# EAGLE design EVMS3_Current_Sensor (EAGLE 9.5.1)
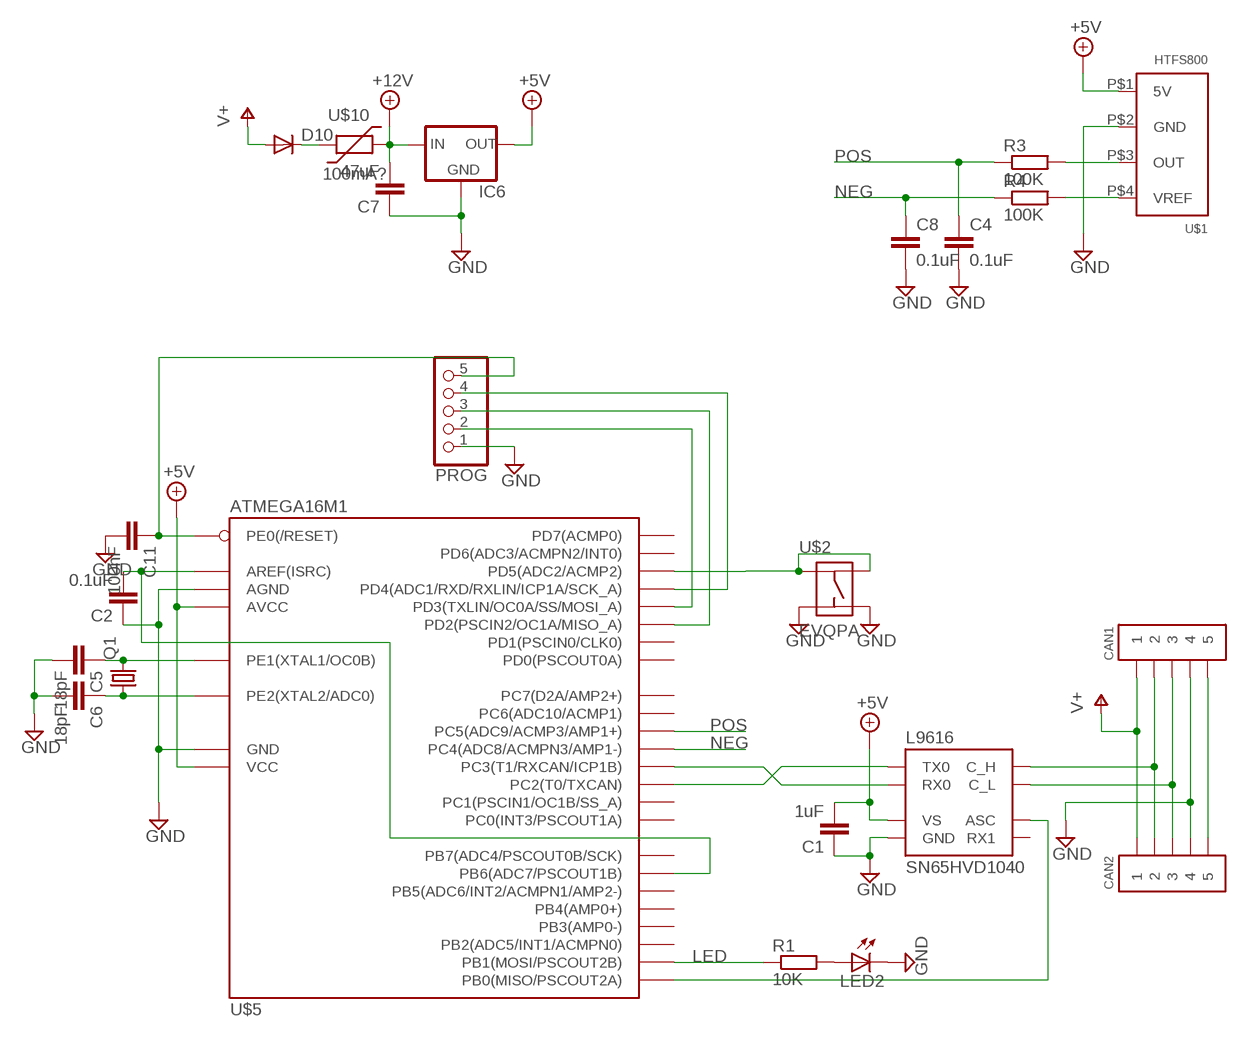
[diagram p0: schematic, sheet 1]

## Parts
C1  1uF  C-EUC1206  [C1206]
C2  0.1uF  C-EUC1206  [C1206]
C4  0.1uF  C-EUC1206  [C1206]
C5  18pF  C-EUC0805  [C0805]
C6  18pF  C-EUC0805  [C0805]
C7  47uF  C-EUC1206  [C1206]
C8  0.1uF  C-EUC1206  [C1206]
C11  100nF  C-EUC1206  [C1206]
CAN1  MOLEX-39502-1005  [MOLEX-39502-1005]
CAN2  MOLEX-39502-1005  [MOLEX-39502-1005]
D10  DIODE-SOD123  [SOD123]
IC6  78LXXSOT89  [SOT89R]
LED2  LED3MM  [LED3MM]
PROG  PINHD-1X5  [1X05]
Q1  CRYSTALCTS406  [CTS406]
R1  10K  R-EU_R1206  [R1206]
R3  100K  R-EU_R1206  [R1206]
R4  100K  R-EU_R1206  [R1206]
SN65HVD1040  L9616  [SOIC8]
U$1  HTFS800  [HTFS800]
U$2  EVQPA  [EVQPA]
U$5  ATMEGA16M1  [TQFP32]
U$10  100mA?  1206_POLYSWITCH  [1206]

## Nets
+5V: C1.2 IC6.2(OUT) SN65HVD1040.P$3(VS) U$1.P$1(5V) U$5.4(VCC) U$5.19(AVCC)
+12V: C7.2 IC6.1(IN) U$10.P$2
BUTTON: U$2.B U$2.B2 U$5.13(PD5(ADC2/ACMP2))
GND: C1.1 C2.1 C4.2 C5.2 C6.2 C7.1 C8.2 C11.2 CAN1.4 CAN2.4 IC6.4(GND) LED2.K(C) PROG.1 SN65HVD1040.P$2(GND) U$1.P$2(GND) U$2.A U$2.A2 U$5.5(GND) U$5.20(AGND)
LED: R1.1 U$5.9(PB1(MOSI/PSCOUT2B))
N$1: LED2.A R1.2
N$2: CAN1.5 CAN2.5
N$3: SN65HVD1040.P$8(ASC) U$5.8(PB0(MISO/PSCOUT2A))
N$4: R3.2 U$1.P$3(OUT)
N$5: R4.2 U$1.P$4(VREF)
N$7: CAN1.2 CAN2.2 SN65HVD1040.P$7(C_H)
N$10: CAN1.3 CAN2.3 SN65HVD1040.P$6(C_L)
N$12: SN65HVD1040.P$1(TX0) U$5.6(PC2(T0/TXCAN))
N$15: D10.C U$10.P$1
N$17: SN65HVD1040.P$4(RX0) U$5.7(PC3(T1/RXCAN/ICP1B))
N$21: C6.1 Q1.1 U$5.11(PE2(XTAL2/ADC0))
N$34: C5.1 Q1.3 U$5.10(PE1(XTAL1/OC0B))
N$42: C2.2 U$5.21(AREF(ISRC)) U$5.27(PB6(ADC7/PSCOUT1B))
N$44: C11.1 PROG.5 U$5.31(PE0(/RESET))
NEG: C8.1 R4.1 U$5.17(PC4(ADC8/ACMPN3/AMP1-))
OUT1: PROG.2 U$5.2(PD3(TXLIN/OC0A/SS/MOSI_A))
OUT2: PROG.3 U$5.1(PD2(PSCIN2/OC1A/MISO_A))
OUT3: PROG.4 U$5.12(PD4(ADC1/RXD/RXLIN/ICP1A/SCK_A))
POS: C4.1 R3.1 U$5.18(PC5(ADC9/ACMP3/AMP1+))
V+: CAN1.1 CAN2.1 D10.A
Unconnected: SN65HVD1040.P$5(RX1) U$5.3(PC1(PSCIN1/OC1B/SS_A)) U$5.14(PD6(ADC3/ACMPN2/INT0)) U$5.15(PD7(ACMP0)) U$5.16(PB2(ADC5/INT1/ACMPN0)) U$5.22(PC6(ADC10/ACMP1)) U$5.23(PB3(AMP0-)) U$5.24(PB4(AMP0+)) U$5.25(PC7(D2A/AMP2+)) U$5.26(PB5(ADC6/INT2/ACMPN1/AMP2-)) U$5.28(PB7(ADC4/PSCOUT0B/SCK)) U$5.29(PD0(PSCOUT0A)) U$5.30(PC0(INT3/PSCOUT1A)) U$5.32(PD1(PSCIN0/CLK0))

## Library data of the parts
C1 C2 C4-C8 C11 = resistor:C-EU: CAPACITOR, European symbol
CAN1 CAN2 = Ians parts:MOLEX-39502-1005
D10 = diode:DIODE-: DIODE
IC6 = v-reg:78LXX: VOLTAGE REGULATOR
LED2 = led:LED: LED
PROG = pinhead:PINHD-1X5: PIN HEADER
Q1 = crystal:CRYSTAL: CRYSTAL
R1 R3 R4 = resistor:R-EU_: RESISTOR, European symbol
SN65HVD1040 = Ians parts:L9616
U$1 = Ians parts:HTFS800
U$2 = Ians parts:EVQPA
U$5 = Ians parts:ATMEGA16M1
U$10 = Ians parts:1206_POLYSWITCH

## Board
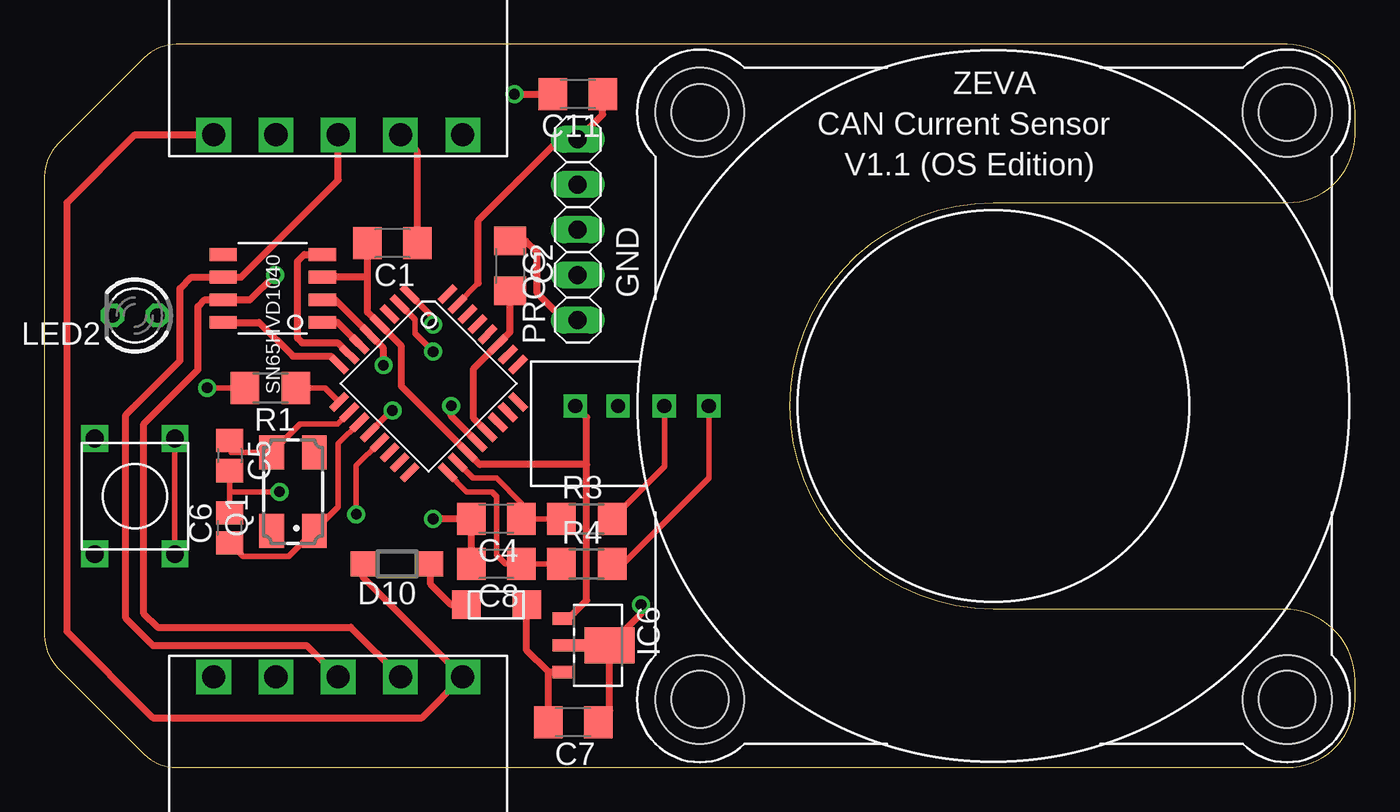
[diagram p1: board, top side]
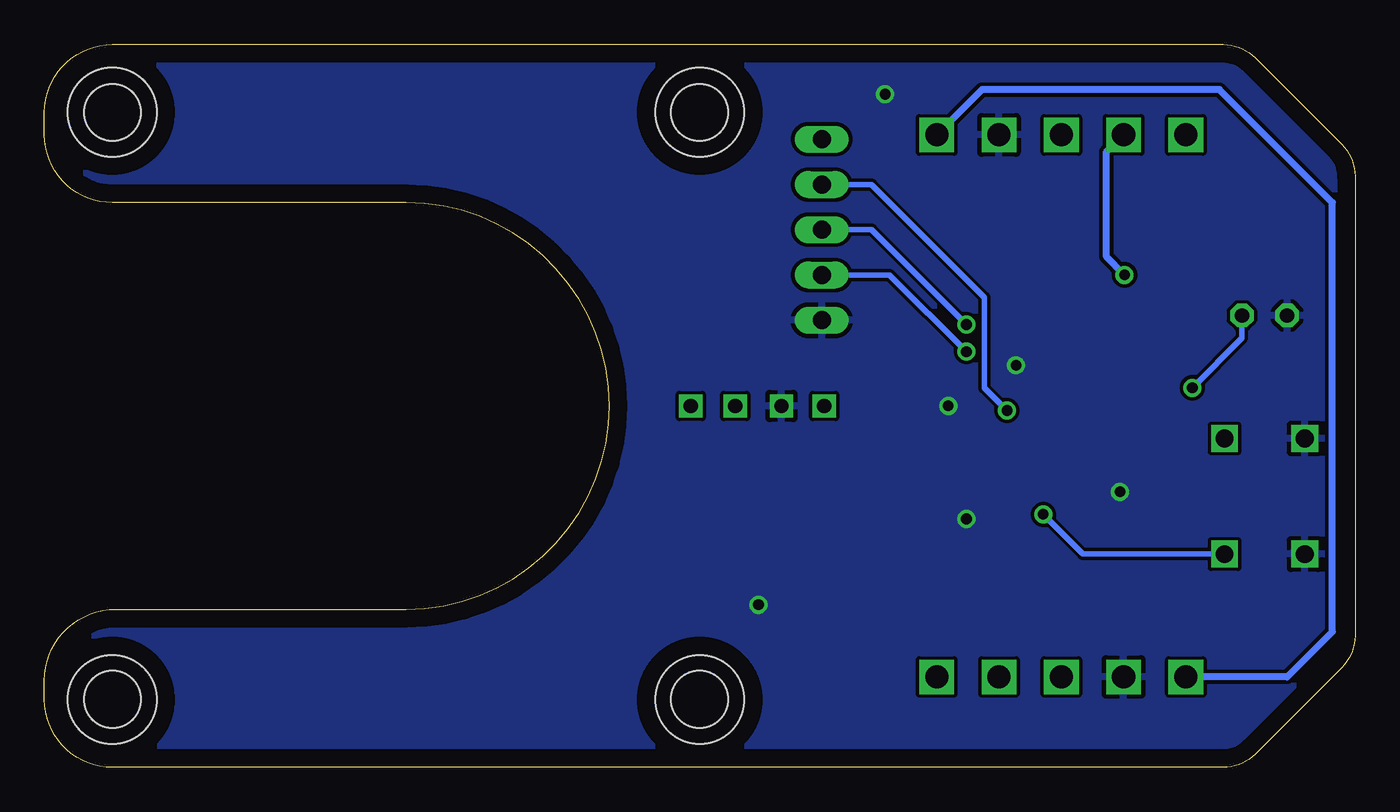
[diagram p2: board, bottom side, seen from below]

Size 73.66 x 40.64 mm. Coordinates in mm from the lower left corner, seen from the top.
Outline: 53.34,8.89 arc-90 41.91,20.32 arc-90 53.34,31.75 69.85,31.75 arc90 73.66,35.56 73.66,36.83 arc90 69.85,40.64 7.4,40.64 arc45 5.61,39.9 0.74,35.03 arc45 0,33.24 0,7.4 arc45 0.74,5.61 5.61,0.74 arc45 7.4,0 69.85,0 arc90 73.66,3.81 73.66,4.87 arc90 69.64,8.89 53.34,8.89
Copper layers (1*16): Top 0.035mm / dielectric 1.5mm / Bottom 0.035mm
Design rules "default *": minimum track width 10mil, minimum drill 20mil, track to track 8mil, track to pad 8mil, pad to pad 8mil, via to via 8mil, smd to smd 8mil, copper to edge 40mil, drill to drill 8mil, minimum pad ring 10mil, minimum via ring 8mil, stop-mask expansion 4mil, vias tented up to drill 0mil, thermal gap 10mil
Holes 5 mm at 36.83,36.83 69.85,36.83 36.83,3.81 69.85,3.81

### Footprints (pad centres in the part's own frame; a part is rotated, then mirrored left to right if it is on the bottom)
C1206 = smd 1.6 x 1.8: 1 -1.4,0; 2 1.4,0
C0805 = smd 1.3 x 1.5: 1 -0.85,0; 2 0.85,0
MOLEX-39502-1005 = drill 1.3 square: 1 -7,0; 2 -3.5,0; 3 0,0; 4 3.5,0; 5 7,0
SOD123 = smd 1.4 x 1.4: A 1.9,0; C -1.9,0
SOT89R = smd 0.7 x 1.1: 1 1.5,-1.75; 2 -1.5,-1.75 | smd 0.7 x 1.8: 3 0,-1.4 | smd 2 x 2.8: 4 0,0.9
LED3MM = drill 0.813 octagon: A -1.27,0; K 1.27,0
1X05 = drill 1.016 long: 1 -5.08,0; 2 -2.54,0; 3 0,0; 4 2.54,0; 5 5.08,0
CTS406 = smd 1.9 x 1.4: 1 -2.2,-1.2; 2 2.2,-1.2; 3 2.2,1.2; 4 -2.2,1.2
R1206 = smd 1.6 x 1.803: 1 -1.422,0; 2 1.422,0
SOIC8 = smd 1.524 x 0.711: P$1 -2.794,1.905; P$2 -2.794,0.635; P$3 -2.794,-0.635; P$4 -2.794,-1.905; P$5 2.794,-1.905; P$6 2.794,-0.635; P$7 2.794,0.635; P$8 2.794,1.905
HTFS800 = drill 0.8 square: P$1 0,-23.5; P$2 0,-21.1; P$3 0,-18.5; P$4 0,-16 | hole 3.2: -16.5,16.5; 16.5,16.5; 16.5,-16.5; -16.5,-16.5
EVQPA = drill 1 square: A -2.25,3.25; A2 -2.25,-3.25; B 2.25,3.25; B2 2.25,-3.25
TQFP32 = smd 1.2 x 0.4: 1 -4.3,2.8; 2 -4.3,2; 3 -4.3,1.2; 4 -4.3,0.4; 5 -4.3,-0.4; 6 -4.3,-1.2; 7 -4.3,-2; 8 -4.3,-2.8; 17 4.3,-2.8; 18 4.3,-2; 19 4.3,-1.2; 20 4.3,-0.4; 21 4.3,0.4; 22 4.3,1.2; 23 4.3,2; 24 4.3,2.8 | smd 0.4 x 1.2: 9 -2.8,-4.3; 10 -2,-4.3; 11 -1.2,-4.3; 12 -0.4,-4.3; 13 0.4,-4.3; 14 1.2,-4.3; 15 2,-4.3; 16 2.8,-4.3; 25 2.8,4.3; 26 2,4.3; 27 1.2,4.3; 28 0.4,4.3; 29 -0.4,4.3; 30 -1.2,4.3; 31 -2,4.3; 32 -2.8,4.3
1206 = smd 1.6 x 1.6: P$1 -1.7,0; P$2 1.7,0

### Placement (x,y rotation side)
C1  19.56,29.46 180 top
C2  26.16,28.19 270 top
C4  25.4,13.97 180 top
C5  10.41,17.53 270 top
C6  10.41,13.46 90 top
C7  29.72,2.54 180 top
C8  25.4,11.43 180 top
C11  29.97,37.85 180 top
CAN1  16.51,35.56 0 top
CAN2  16.51,5.08 180 top
D10  19.81,11.43 180 top
IC6  30.86,6.86 270 top
LED2  5.08,25.4 180 top
PROG  29.97,30.23 90 top
Q1  13.97,15.49 90 top
R1  12.7,21.34 180 top
R3  30.48,13.97 0 top
R4  30.48,11.43 0 top
SN65HVD1040  12.83,26.92 180 top
U$1  53.34,20.32 270 top
U$2  5.08,15.24 0 top
U$5  21.59,21.59 315 top
U$10  25.4,9.14 0 top

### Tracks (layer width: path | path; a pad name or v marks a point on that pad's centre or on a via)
+5V
  Top 0.406: IC6.2 29.44,8.36 30.48,9.4 30.48,17.02 | 30.48,17.02 30.48,19.68 U$1.P$1 | 30.48,17.02 24.46,17.02 U$5.19 20.07,21.42 20.07,23.68 U$5.4 18.16,25.59 18.16,27.56 | 18.16,27.56 C1.2 | 18.16,27.56 SN65HVD1040.P$3
+12V
  Top 0.406: 28.76,5.46 IC6.1 28.32,5.36 | C7.2 28.32,5.36 | U$10.P$2 27.1,6.58 28.32,5.36
BUTTON  (via drill 0.6)
  Top 0.305: U$2.B2 U$2.B | U$5.13 17.53,16.96 v17.53,14.22
  Bottom 0.305: U$2.B2 15.29,11.99 v17.53,14.22
GND  (via drill 0.6)
  Top 0.305: C6.2 10.41,15.49 | 10.41,15.49 C5.2 | 10.41,15.49 v13.21,15.49
  Top 0.406: v21.84,13.97 C4.2 C8.2 | U$5.20 22.86,19.75 v22.86,20.32 | v19.05,22.61 19.05,23.56 U$5.5 16.32,26.29 SN65HVD1040.P$2 | C2.1 27.05,29.59 27.69,28.96 27.69,26.67 29.21,25.15 PROG.1 | v26.42,37.85 C11.2 | C1.1 20.96,34.61 CAN1.4 | C7.1 31.76,3.18 IC6.4 33.53,8.62 v33.53,9.14
  pour Bottom: -1.27,-0.64 74.93,-0.64 74.93,41.27 -1.27,41.27
LED
  Top 0.305: R1.1 15.76,21.34 U$5.9
N$1  (via drill 0.6)
  Top 0.305: v9.14,21.34 R1.2
  Bottom 0.305: LED2.A 6.35,24.13 v9.14,21.34
N$2
  Bottom 0.406: CAN2.5 3.81,5.08 1.27,7.62 1.27,31.75 7.62,38.1 20.97,38.1 CAN1.5
N$3
  Top 0.406: U$5.8 16.11,23.11 13.97,23.11 12.06,25.02 SN65HVD1040.P$8
N$4
  Top 0.305: U$1.P$3 34.84,16.91 R3.2
N$5
  Top 0.305: U$1.P$4 37.34,16.26 32.51,11.43 R4.2
N$7  (via drill 0.6)
  Top 0.406: v12.95,27.69 11.56,26.29 SN65HVD1040.P$7 9.02,26.29 8.64,25.91 8.64,22.35 5.59,19.3 5.59,8.64 6.35,7.87 17.22,7.87 CAN2.2
  Bottom 0.406: v12.95,27.69 13.97,28.7 13.97,34.6 CAN1.2
N$10
  Top 0.406: CAN1.3 16.51,33.02 11.05,27.56 SN65HVD1040.P$6 8.26,27.56 7.62,26.92 7.62,22.86 4.57,19.81 4.57,8.38 6.1,6.86 14.73,6.86 CAN2.3
N$12
  Top 0.406: SN65HVD1040.P$1 16.46,25.02 U$5.6
N$15
  Top 0.406: D10.C 21.71,10.29 22.86,9.14 U$10.P$1
N$17
  Top 0.406: U$5.7 16.48,23.88 14.48,23.88 14.22,24.13 14.22,28.45 14.61,28.83 SN65HVD1040.P$4
N$21
  Top 0.305: U$5.11 16.51,18.21 16.51,14.63 Q1.1 13.73,11.85 11.18,11.85 C6.1
N$34
  Top 0.305: U$5.10 16.48,19.3 14.38,19.3 Q1.3 10.49,17.69 C5.1
N$42
  Top 0.406: U$5.21 24.13,19.62 24.13,22.43 U$5.27 26.16,24.46 C2.2
N$44
  Top 0.305: U$5.31 24.38,27.21
  Top 0.406: 24.38,27.21 24.38,30.73 28.96,35.31 PROG.5 31.37,36.71 C11.1
NEG
  Top 0.305: R4.1 C8.1 25.91,11.43 25.4,11.94 25.4,15.24 25.15,15.49 23.73,15.49 U$5.17
OUT1  (via drill 0.6)
  Top 0.305: U$5.2 20.83,25.18 20.83,24.38 v21.84,23.37
  Bottom 0.305: PROG.2 26.16,27.69 v21.84,23.37
OUT2  (via drill 0.6)
  Top 0.305: U$5.1 21.84,25.3 v21.84,24.89
  Bottom 0.305: PROG.3 27.18,30.23 v21.84,24.89
OUT3  (via drill 0.6)
  Top 0.305: v19.56,20.07 19.5,20.07 U$5.12
  Bottom 0.305: PROG.4 27.18,32.77 20.83,26.42 20.83,21.34 v19.56,20.07
POS
  Top 0.305: R3.1 C4.1 26.8,14.86 25.4,16.26 24.1,16.26 U$5.18
V+
  Top 0.406: CAN1.1 5.08,35.56 1.27,31.75 1.27,7.62 6.1,2.79 21.22,2.79 CAN2.1 17.91,10.68 D10.A

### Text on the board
tPlace: ZEVA | CAN Current Sensor | V1.1 (OS Edition) | GND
